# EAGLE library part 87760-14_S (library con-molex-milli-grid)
HEADER
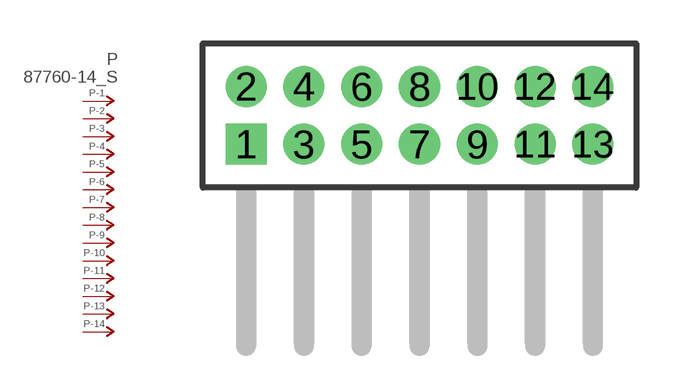
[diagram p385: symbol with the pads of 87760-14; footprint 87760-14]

Designator prefix P; gates -1=P-NV -2=P-N -3=P-N -4=P-N -5=P-N -6=P-N -7=P-N -8=P-N -9=P-N -10=P-N -11=P-N -12=P-N -13=P-N -14=P-N

## 87760-14_S  [87760-14]
1  -1:P  pas
2  -2:P  pas
3  -3:P  pas
4  -4:P  pas
5  -5:P  pas
6  -6:P  pas
7  -7:P  pas
8  -8:P  pas
9  -9:P  pas
10  -10:P  pas
11  -11:P  pas
12  -12:P  pas
13  -13:P  pas
14  -14:P  pas

## Footprint 87760-14 (pad centres in mm)
HEADER Dual Row, Right Angle
drill 0.914 square: 1 -6,-1
drill 0.914: 2 -6,1; 3 -4,-1; 4 -4,1; 5 -2,-1; 6 -2,1; 7 0,-1; 8 0,1; 9 2,-1; 10 2,1; 11 4,-1; 12 4,1; 13 6,-1; 14 6,1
